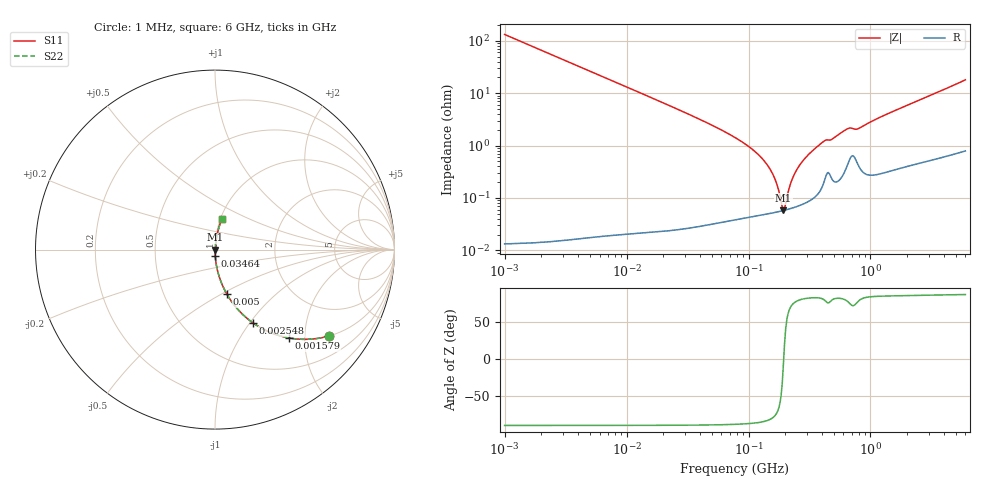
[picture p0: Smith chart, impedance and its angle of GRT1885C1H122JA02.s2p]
!Murata Part Number: GRT1885C1H122JA02
!These Parameters are Measured in Series Mode Connection
!Data Generated on Jun 19, 2026
!  o--ll--o
!Port1  Port2
!  o------o
!Operation Temp=25[degC], DC Bias Voltage=0[V]
!Freq. Start=1000[kHz] Stop=6[GHz] 401[Steps]
# Hz S RI R 50
!Freq.(Hz) S11(Real) S11(Imag) S21(Real) S21(Imag) S12(Real) S12(Imag) S22(Real) S22(Imag)
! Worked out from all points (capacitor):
!   401 points, 1 MHz to 6 GHz, reference 50 ohm
!   read as one part in series: C = 1.2 nF near 1.044 MHz
!   lowest |Z| = 58.1 mohm at 193.1 MHz (marker M1)
!   series resonance near 194.2 MHz, so ESL is about 560 pH
!   S11 on the Smith chart (normalised r, x): 1 MHz: 1.00, -2.64; 1.579 MHz: 1.00, -1.67; 2.548 MHz: 1.00, -1.04; 5 MHz: 1.00, -0.53; 34.64 MHz: 1.00, -0.07; 6 GHz: 1.02, +0.36
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1000000  0.6361 -0.4811  0.3639 0.4811  0.3639 0.4811  0.6361 -0.4811
1578894  0.4122 -0.4921  0.5878 0.4921  0.5878 0.4921  0.4122 -0.4921
2547717  0.2122 -0.4087  0.7878 0.4087  0.7878 0.4087  0.2122 -0.4087
4293785  0.0866 -0.281  0.9134 0.281  0.9134 0.281  0.0866 -0.281
4999862  0.0654 -0.2469  0.9346 0.2469  0.9346 0.2469  0.0654 -0.2469
1.843659e7  0.00524 -0.0706  0.9948 0.0706  0.9948 0.0706  0.00524 -0.0706
3.46415e7  0.00163 -0.0368  0.9984 0.0368  0.9984 0.0368  0.00163 -0.0368
7.745967e7  0.000585 -0.0143  0.9994 0.0143  0.9994 0.0143  0.000585 -0.0143
1.121107e8  0.000507 -0.0078  0.9995 0.0078  0.9995 0.0078  0.000507 -0.0078
1.424119e8  0.000512 -0.00426  0.9995 0.00426  0.9995 0.00426  0.000512 -0.00426
1.658303e8  0.000535 -0.00214  0.9995 0.00214  0.9995 0.00214  0.000535 -0.00214
1.848803e8  0.000563 -0.000665  0.9994 0.000665  0.9994 0.000665  0.000563 -0.000665
1.930997e8  0.000576 -7.57e-05  0.9994 7.57e-05  0.9994 7.57e-05  0.000576 -7.57e-05
2.016844e8  0.000592 0.000514  0.9994 -0.000514  0.9994 -0.000514  0.000592 0.000514
2.200158e8  0.000629 0.0017  0.9994 -0.0017  0.9994 -0.0017  0.000629 0.0017
2.452905e8  0.000688 0.00321  0.9993 -0.00321  0.9993 -0.00321  0.000688 0.00321
3.325952e8  0.00101 0.0078  0.999 -0.0078  0.999 -0.0078  0.00101 0.0078
4.133993e8  0.00208 0.0119  0.9979 -0.0119  0.9979 -0.0119  0.00208 0.0119
6.386712e8  0.00432 0.02  0.9957 -0.02  0.9957 -0.02  0.00432 0.02
7.938365e8  0.00463 0.0205  0.9954 -0.0205  0.9954 -0.0205  0.00463 0.0205
1.428092e9  0.00493 0.0414  0.9951 -0.0414  0.9951 -0.0414  0.00493 0.0414
6e9  0.0386 0.172  0.9614 -0.172  0.9614 -0.172  0.0386 0.172
